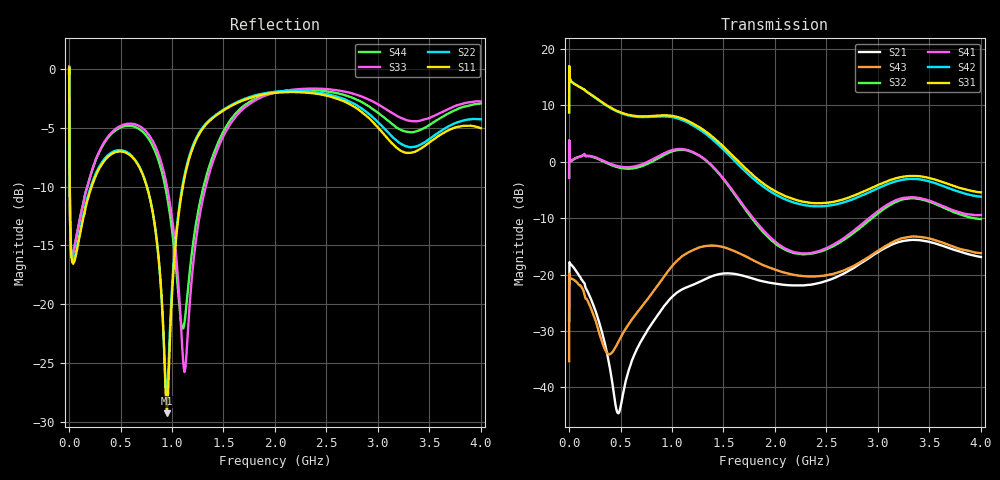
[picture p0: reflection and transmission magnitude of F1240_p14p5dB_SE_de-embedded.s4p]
! Integrated Device Technology
! Corporate Headquarters
! 6024 Silver Creek Valley Road
! San Jose, CA 95138  USA
! Phone:  1-408-284-8200
! Toll Free:  1-800-223-1366
! Webpage:  http://www.idt.com/
! Timing and RF Division
! 515 Groton Road, Suite 102
! Westford, MA 01886-6024
! Device:  F1240
! Description: Dual Intermediate Frequency Digital Variable Gain Amplifier
! Frequency:  10.0 -  500.00 MHz
! Package:  5x5 mm QFN Plastic Package: 32 pin
! Ports:  8 RF, 20 DC
!  Pin  1  = GA3 / Data  Pin 17  = RF OUT_B+
!  Pin  2  = GA4 / CLK  Pin 18  = RF OUT_B-
!  Pin  3  = GA5  Pin 19  = STBY_B
!  Pin  4  = VMODE  Pin 20  = Ground
!  Pin  5  = No Connect  Pin 21  = Ground
!  Pin  6  = GB5  Pin 22  = STB_A
!  Pin  7  = GB4  Pin 23  = RF OUT_A-  = Port 4
!  Pin  8  = GB3  Pin 24  = RF OUT_A+  = Port 3
!  Pin  9  = GB2  Pin 25  = GA0
!  Pin 10  = GB1  Pin 26  = ISET_A
!  Pin 11  = RF IN_B+  Pin 27  = VCC
!  Pin 12  = RF IN_B-  Pin 28  = Ground
!  Pin 13  = Ground  Pin 29  = RF IN_A-  = Port 2
!  Pin 14  = VCC  Pin 30  = RF IN_A+  = Port 1
!  Pin 15  = ISET_B  Pin 31  = GA1
!  Pin 16  = GB0  Pin 32  = GA2 / CSb
! Gain  = +19.5 dB
! State  = 1
! Voltage  = +5.00 V
! Current  = 85.292 mA (one channel only)
! Temperture  =  +25 C
! Test Date  =  2017-10-18
! Board  =  EB4031
! Data:  The device was measured on a custom evaluation board which has
!  individual transmission lines to the RF pins.  Data was collected
!  using a calibrated network analyzer.  The evaluation board was
!  de-embedded using Automatic Fixture Removal.
!  The reference plane is the edge of the package pin.
!  Only Channel A was measured.
!  This data is in single-ended operation.  If your needs are balanced
!  or differential S-parameters then this file needs to be used a
!  linear simulator.
! File Date:  2017-11-10  MJV
! Note:
!  Integrated Device Technology supplies this data as a sample of measured
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# Hz S dB R 100
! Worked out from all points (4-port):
!   410 points, 500 kHz to 4 GHz, reference 100 ohm
!   strongest paths, dB at 500 kHz, 930 MHz, 1.96 GHz, 2.98 GHz, 4 GHz:
!     S31: 8.8, 8.3, -4.7, -4.3, -5.4
!     S42: 8.8, 8.1, -5.3, -4.9, -6.2
!     S41: -2.9, 1.6, -13.5, -9.1, -9.4
!     S32: -2.8, 1.3, -13.8, -9.4, -10.1
!     S43: -35.4, -20.2, -18.9, -16.0, -16.2
!     S21: -28.2, -25.4, -21.5, -16.3, -16.9
!   lowest |S11| = -29.3 dB at 950 MHz (marker M1), VSWR 1.07, Z = 106 + j3.52 ohm
!   |S11| at or under -10 dB: 6.989 MHz to 219.4 MHz (212.4 MHz wide, 188 % of centre); 755.6 MHz to 1.105 GHz (349.4 MHz wide, 37.6 % of centre)
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500000  -0.33 -6.1  -28.10 4.0  -27.31 77.4  -60.28 65.6
        -28.17 3.8  -0.33 -6.0  -60.33 65.0  -27.32 78.5
        8.80 -105.3  -2.84 72.1  -0.43 1.1  -35.40 -150.6
        -2.85 73.1  8.78 -104.1  -35.38 -150.9  -0.44 3.4
3000000  -4.30 -57.0  -18.01 16.2  -18.51 15.5  -39.70 60.4
         -18.00 16.1  -4.26 -57.1  -39.64 60.5  -18.52 15.6
         16.34 -174.1  2.11 -7.7  -3.88 -52.7  -19.84 38.2
         2.11 -7.6  16.34 -173.9  -19.81 38.1  -3.94 -52.5
2e8  -10.52 -119.0  -23.75 -96.1  -21.16 -51.3  -34.24 8.0
     -23.79 -95.0  -10.32 -120.5  -34.23 8.3  -21.18 -51.3
     12.12 109.8  0.98 -51.3  -9.29 -82.6  -24.96 -105.4
     1.06 -51.3  12.08 109.0  -25.45 -103.1  -9.29 -81.8
5.4e8  -7.06 -174.6  -39.67 47.2  -22.84 -108.3  -28.11 -58.5
       -39.82 30.6  -6.97 -175.9  -28.24 -57.0  -22.99 -108.6
       8.53 24.7  -1.19 -128.1  -4.69 -152.0  -31.10 57.9
       -0.94 -129.3  8.43 23.7  -29.89 36.8  -4.84 -151.7
9.5e8  -29.30 28.9  -23.68 -58.0  -20.35 167.8  -23.64 -155.1
       -25.00 -67.9  -28.10 21.1  -23.95 -150.2  -20.75 167.2
       8.24 -75.8  1.46 141.4  -9.93 143.7  -20.50 -41.2
       1.74 136.8  8.05 -77.6  -19.66 -59.1  -10.74 147.5
1.52e9  -3.39 -147.1  -19.52 155.3  -26.13 34.3  -25.76 70.7
        -19.79 160.0  -3.33 -147.2  -25.62 76.5  -27.29 33.1
        2.34 122.6  -3.57 -41.8  -5.34 -130.7  -15.43 146.8
        -3.44 -46.8  1.81 121.2  -15.24 140.6  -4.97 -134.1
4e9  -5.02 -156.0  -16.93 62.6  -21.42 -46.5  -19.84 -48.4
     -16.88 61.9  -4.26 -150.5  -22.10 -29.4  -24.71 -34.4
     -5.42 7.2  -10.15 -120.5  -2.74 -137.0  -15.46 89.7
     -9.44 -131.6  -6.18 16.3  -16.21 62.9  -2.91 -142.6
